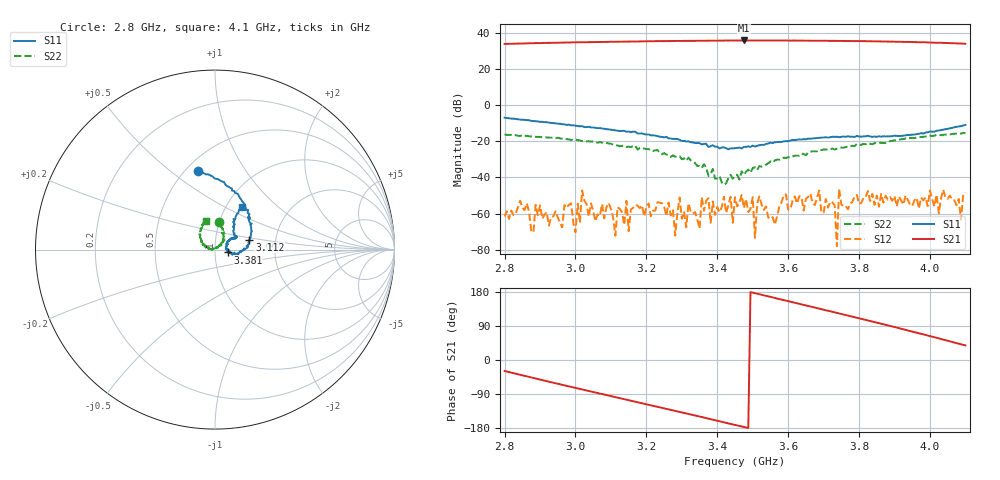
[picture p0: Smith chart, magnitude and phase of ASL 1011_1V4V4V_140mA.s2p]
!ASL 1011 Low Noise Amplifier
!Test-Fixture S-parameter data in 2.8-4 GHz
!Bias conditions Vd1=1V,Vd2=4V,Vd3=4V ; Ids =140mA
!freq-unit  param-type  data-format  keyword  impedance-ohms
# GHz  S  DB  R  50
!Freq  DBS11  AngS11  DBS21  AngS21  DBS12  AngS12  DBS22  AngS22
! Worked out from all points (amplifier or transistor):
!   209 points, 2.8 GHz to 4.1 GHz, reference 50 ohm
!   highest |S21| = 35.7 dB at 3.475 GHz (marker M1)
!   |S21| within 3 dB of that: start of sweep to end of sweep
!   unconditionally stable (mu >= 1): start of sweep to end of sweep
!   at 3.013 GHz: K = 15.27, MAG = 35.0 dB, |S12| = -65.0 dB
!   at 3.45 GHz: K = 2.98, MAG = 35.7 dB, |S12| = -51.0 dB
!   at 4.1 GHz: K = 2.49, MAG = 34.3 dB, |S12| = -48.3 dB
!   S11 on the Smith chart (normalised r, x): 2.8 GHz: 0.58, +0.63; 3.112 GHz: 1.46, +0.17; 3.381 GHz: 1.15, -0.04; 4.1 GHz: 1.18, +0.61
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2.8  -7.02 102.2  33.75 -29.0  -61.57 -28.2  -16.20 82.6
2.9063  -9.28 71.7  34.27 -53.0  -62.85 -117.0  -17.75 74.7
3.0187  -11.71 44.7  34.71 -77.7  -47.17 3.5  -19.94 67.9
3.1125  -14.02 16.1  34.98 -98.0  -72.23 8.3  -22.18 53.6
3.175  -15.76 -0.3  35.14 -111.3  -55.58 -117.9  -24.66 44.8
3.2375  -17.48 -9.1  35.33 -124.8  -54.00 91.2  -26.57 47.6
3.3062  -19.82 -13.8  35.46 -139.6  -59.08 134.7  -29.48 43.8
3.3813  -22.77 -12.6  35.58 -156.2  -65.09 15.4  -38.11 39.5
3.45  -23.85 8.8  35.67 -171.4  -50.95 114.6  -39.19 145.9
3.475  -23.17 18.9  35.68 -176.8  -56.87 128.4  -38.59 162.8
3.5625  -20.61 33.9  35.65 163.8  -66.15 58.0  -30.62 173.4
3.6125  -19.27 35.2  35.63 152.6  -52.73 136.5  -28.44 167.4
3.6688  -18.50 32.9  35.54 139.8  -54.01 54.6  -25.55 161.4
3.7062  -17.81 28.8  35.49 131.1  -51.99 38.8  -24.64 161.2
3.7375  -17.54 30.3  35.42 124.4  -78.01 48.8  -24.07 159.6
3.7437  -17.80 28.6  35.44 123.0  -46.40 37.4  -23.82 154.0
3.7875  -17.66 30.0  35.34 113.0  -50.55 38.4  -22.71 157.4
3.8875  -17.32 38.6  35.02 89.8  -50.88 18.5  -19.92 142.1
3.9375  -16.57 45.4  34.90 78.0  -52.43 -3.1  -18.52 134.1
3.9813  -15.81 50.7  34.68 67.6  -52.75 24.2  -17.57 126.5
4.0375  -13.58 56.8  34.34 53.7  -46.81 -10.0  -16.47 117.7
4.1  -10.98 57.9  33.87 38.4  -48.34 -8.5  -15.48 108.3
